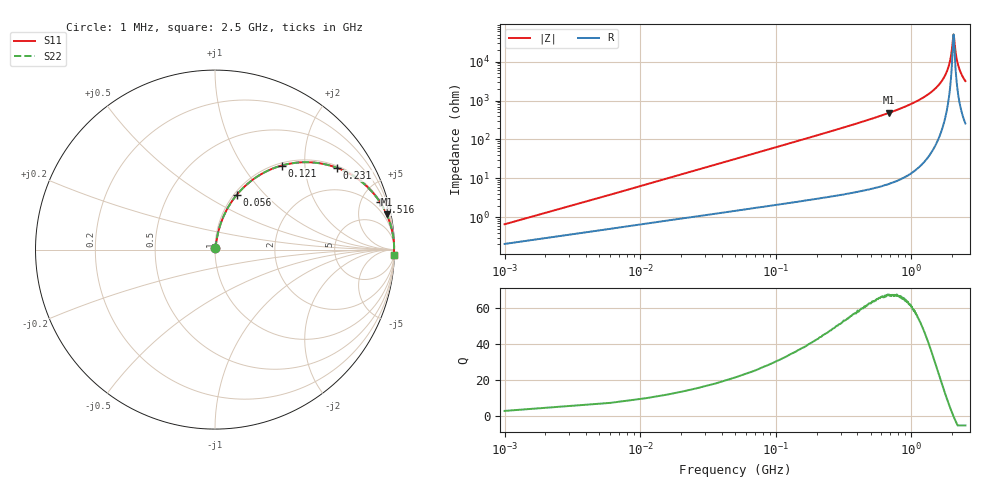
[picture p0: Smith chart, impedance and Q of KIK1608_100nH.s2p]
!version-2
!date-01.2022
!Series
# MHz S RI R 50
!Freq ReS11 ImS11 ReS21 ImS21 ReS12 ImS12 ReS22 ImS22
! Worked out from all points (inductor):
!   501 points, 1 MHz to 2.5 GHz, reference 50 ohm
!   read as one part in series: L = 100 nH near 11 MHz
!   highest Q = 67 at 686 MHz (marker M1), where L = 113 nH
!   self-resonance near 2.045 GHz
!   S11 on the Smith chart (normalised r, x): 1 MHz: 1.00, +0.01; 56 MHz: 1.03, +0.70; 121 MHz: 1.05, +1.53; 231 MHz: 1.06, +2.94; 516 MHz: 1.11, +6.92; 2.5 GHz: 6, -63
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1  0.0021 0.00626  0.9979 -0.00626  0.9979 -0.00626  0.0021 0.00626
16  0.018 0.0979  0.982 -0.0979  0.982 -0.0979  0.018 0.0979
21  0.026 0.1273  0.974 -0.1273  0.974 -0.1273  0.026 0.1273
36  0.0592 0.2102  0.9408 -0.2102  0.9408 -0.2102  0.0592 0.2102
56  0.1209 0.3048  0.8791 -0.3048  0.8791 -0.3048  0.1209 0.3048
121  0.3718 0.4685  0.6282 -0.4685  0.6282 -0.4685  0.3718 0.4685
231  0.6801 0.4556  0.3199 -0.4556  0.3199 -0.4556  0.6801 0.4556
421  0.88 0.3166  0.12 -0.3166  0.12 -0.3166  0.88 0.3166
516  0.9195 0.2643  0.0805 -0.2643  0.0805 -0.2643  0.9195 0.2643
686  0.9566 0.1964  0.0434 -0.1964  0.0434 -0.1964  0.9566 0.1964
836  0.9732 0.154  0.0267 -0.154  0.0267 -0.154  0.9732 0.154
1255  0.9921 0.0782  0.00788 -0.0782  0.00788 -0.0782  0.9921 0.0782
1670  0.9973 0.0316  0.00272 -0.0316  0.00272 -0.0316  0.9973 0.0316
1810  0.9978 0.019  0.00216 -0.019  0.00216 -0.019  0.9978 0.019
1910  0.998 0.0106  0.00198 -0.0106  0.00198 -0.0106  0.998 0.0106
1975  0.998 0.00543  0.00196 -0.00543  0.00196 -0.00543  0.998 0.00543
2040  0.998 0.000414  0.00199 -0.000414  0.00199 -0.000414  0.998 0.000414
2055  0.998 -0.00072  0.002 0.00072  0.002 0.00072  0.998 -0.00072
2085  0.998 -0.00296  0.00204 0.00296  0.00204 0.00296  0.998 -0.00296
2145  0.9979 -0.00736  0.00215 0.00736  0.00215 0.00736  0.9979 -0.00736
2225  0.9976 -0.013  0.00236 0.013  0.00236 0.013  0.9976 -0.013
2500  0.9965 -0.0311  0.00352 0.0311  0.00352 0.0311  0.9965 -0.0311
